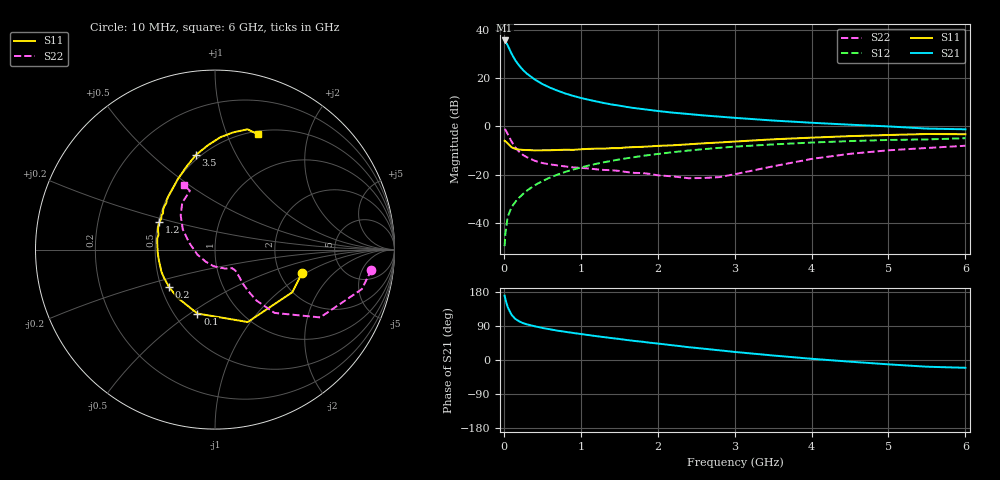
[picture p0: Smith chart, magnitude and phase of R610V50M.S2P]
! SIEMENS Small Signal Semiconductors
! BFR193
! Si NPN RF Bipolar Junction Transistor in SOT23
! VCE = 10 V  IC = 50 mA
! Common Emitter S-Parameters:  May  1996
# GHz  S  MA  R  50
!  f  S11  S21  S12  S22
! GHz  MAG  ANG  MAG  ANG  MAG  ANG  MAG  ANG
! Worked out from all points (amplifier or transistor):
!   36 points, 10 MHz to 6 GHz, reference 50 ohm
!   highest |S21| = 35.6 dB at 10 MHz (marker M1)
!   |S21| within 3 dB of that: start of sweep to 64.12 MHz
!   unconditionally stable (mu >= 1): 441.9 MHz to 2.221 GHz
!   at 250 MHz: K = 0.93, MSG = 25.6 dB, |S12| = -28.0 dB
!   at 1.4 GHz: K = 1.02, MAG = 10.7 dB, |S12| = -14.3 dB
!   at 6 GHz: K = 0.95, MSG = 1.8 dB, |S12| = -4.9 dB
!   S11 on the Smith chart (normalised r, x): 10 MHz: 2.65, -0.92; 100 MHz: 0.65, -0.53; 200 MHz: 0.55, -0.25; 1.2 GHz: 0.51, +0.17; 3.5 GHz: 0.47, +0.70; 6 GHz: 0.54, +1.30
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0.01  0.5027 -15.0  60.01 169.8  0.0033 69.6  0.8787 -7.3
0.02  0.4917 -28.9  57.77 160.7  0.006 70.5  0.8469 -15.1
0.05  0.4428 -65.7  47.47 139.5  0.0133 67.9  0.6974 -32.8
0.1  0.3694 -105.4  32.05 119.3  0.0212 65.2  0.485 -46.7
0.15  0.3397 -128.1  23.21 108.3  0.0273 66.1  0.3646 -50.9
0.2  0.3298 -141.2  18.05 101.9  0.0335 68.0  0.2977 -51.3
0.25  0.3249 -151.0  14.64 97.3  0.0399 69.4  0.2547 -50.9
0.3  0.3229 -157.6  12.32 94.1  0.0467 70.7  0.2288 -49.9
0.4  0.3182 -168.8  9.389 89.1  0.0599 72.2  0.1941 -47.8
0.5  0.3193 -175.8  7.53 84.7  0.0734 72.2  0.174 -46.2
0.6  0.3202 178.8  6.323 81.0  0.0869 71.6  0.1632 -45.9
0.7  0.3237 173.8  5.457 77.4  0.1003 71.2  0.1551 -46.1
0.8  0.3277 169.1  4.784 74.4  0.1141 70.1  0.1477 -47.0
1.1  0.3415 157.8  3.556 65.8  0.154 66.9  0.1342 -51.6
1.2  0.3448 153.9  3.285 63.0  0.1673 65.7  0.1288 -53.6
1.6  0.3669 141.8  2.517 52.7  0.2181 60.2  0.113 -66.2
2.2  0.4053 127.2  1.918 38.7  0.2919 51.6  0.0918 -96.4
2.8  0.4631 113.5  1.59 25.6  0.3586 42.5  0.0888 -148.8
3.5  0.5387 101.3  1.319 11.9  0.4224 31.6  0.1486 165.2
4.5  0.6267 87.3  1.081 -4.4  0.4955 17.9  0.2698 135.1
5.5  0.6941 74.9  0.898 -17.7  0.5352 4.5  0.3562 113.1
6  0.6856 69.3  0.868 -20.6  0.5681 0.7  0.3962 115.6
